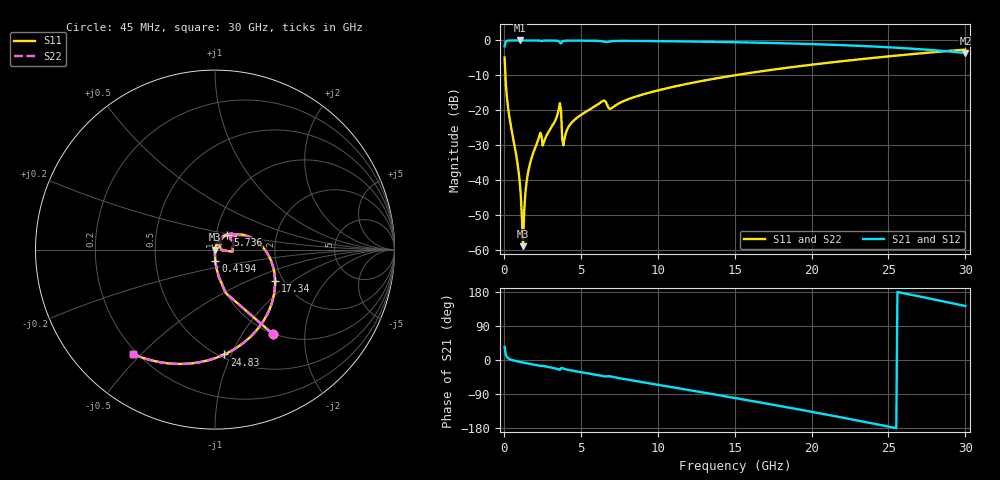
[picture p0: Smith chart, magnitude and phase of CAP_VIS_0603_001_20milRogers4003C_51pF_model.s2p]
! S-parameter model data by Modelithics Inc.  support@modelithics.com  813-866-6335  Tampa FL USA
! S-Parameter data specifications:
! Substrate: 20-mil Rogers 4003C, substrate thickness, H=0.508mm, Dielectric constant, Er=3.75
! PCB Mounting Pad Footprint: Pad width, PadW=0.90mm , Pad length, PadL=1.00mm , Pad gap, PadG (edge-to-edge)=1.00mm , Reference planes=3.0mm apart
! Created Wed Nov 18 13:29:13 2015
# hz S ma R 50
! 2 Port Network Data from SP1.SP block
! freq  magS11  angS11  magS21  angS21  magS12  angS12  magS22  angS22
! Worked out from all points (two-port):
!   401 points, 45 MHz to 30 GHz, reference 50 ohm
!   highest |S21| = -0.01 dB at 1.019 GHz (marker M1); lowest = -3.6 dB at 30 GHz (marker M2)
!   |S21| within 3 dB of the highest: start of sweep to 28.55 GHz
!   lowest |S11| = -58.9 dB at 1.243 GHz (marker M3), VSWR 1.00, Z = 50.1 + j0.0299 ohm
!   |S11| at or under -10 dB: 98.09 MHz to 14.99 GHz (14.89 GHz wide, 197 % of centre)
!   |S22| runs from -58.9 to -2.6 dB; largest |S21 - S12| = 0
!   S11 on the Smith chart (normalised r, x): 45 MHz: 0.99, -1.38; 419.4 MHz: 1.00, -0.13; 5.736 GHz: 1.13, +0.19; 17.34 GHz: 1.81, -0.74; 24.83 GHz: 0.53, -0.94; 30 GHz: 0.18, -0.47
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4.5e7  0.5677 -55.6  0.823 34.3  0.823 34.3  0.5677 -55.6
4.194375e8  0.0655 -88.0  0.9972 1.5  0.9972 1.5  0.0655 -88.0
8.687625e8  0.0182 -90.9  0.9989 -3.7  0.9989 -3.7  0.0182 -90.9
1.018538e9  0.009867 -89.5  0.9989 -5.0  0.9989 -5.0  0.009867 -89.5
1.093425e9  0.006245 -86.6  0.9989 -5.6  0.9989 -5.6  0.006245 -86.6
1.2432e9  0.001131 15.3  0.9988 -6.8  0.9988 -6.8  0.001131 15.3
1.318088e9  0.003619 65.2  0.9988 -7.4  0.9988 -7.4  0.003619 65.2
1.54275e9  0.01189 75.2  0.9986 -9.1  0.9986 -9.1  0.01189 75.2
1.692525e9  0.01712 75.5  0.9984 -10.2  0.9984 -10.2  0.01712 75.5
2.291625e9  0.04164 68.8  0.9943 -14.8  0.9943 -14.8  0.04164 68.8
2.666062e9  0.0386 67.6  0.9952 -16.7  0.9952 -16.7  0.0386 67.6
3.564712e9  0.1034 51.9  0.9715 -25.1  0.9715 -25.1  0.1034 51.9
3.93915e9  0.03912 51.6  0.9889 -23.5  0.9889 -23.5  0.03912 51.6
5.062462e9  0.08727 55.6  0.9928 -32.5  0.9928 -32.5  0.08727 55.6
5.73645e9  0.1076 50.6  0.9896 -37.3  0.9896 -37.3  0.1076 50.6
1.007992e10  0.1941 23.1  0.9766 -65.8  0.9766 -65.8  0.1941 23.1
1.50225e10  0.3171 -11.0  0.9431 -100.3  0.9431 -100.3  0.3171 -11.0
1.734401e10  0.3776 -27.6  0.9201 -117.0  0.9201 -117.0  0.3776 -27.6
2.003996e10  0.4501 -47.5  0.8863 -137.0  0.8863 -137.0  0.4501 -47.5
2.483276e10  0.5863 -84.9  0.8017 -174.4  0.8017 -174.4  0.5863 -84.9
2.505742e10  0.5929 -86.7  0.7967 -176.2  0.7967 -176.2  0.5929 -86.7
3e10  0.7392 -128.0  0.6625 142.5  0.6625 142.5  0.7392 -128.0
